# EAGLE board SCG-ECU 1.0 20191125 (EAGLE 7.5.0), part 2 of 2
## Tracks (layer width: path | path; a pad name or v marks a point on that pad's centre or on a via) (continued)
N$3 (continued)
  Top 0.61: R67.1 79.63,102.01 80.16,101.47 80.16,100.03 U$9.5
N$4  (via drill 0.5)
  other vias: 11.05,95
N$5
  Top 0.61: R68.1 76.86,102.23 77.57,101.52 77.57,100.03 U$9.7
N$6
  Top 0.61: R35.1 64.54,101.91 65.02,101.42 U$11.5
N$7  (via drill 0.5)
  other vias: 12.32,95
N$8
  Top 0.61: R36.1 61.85,102.16 62.48,101.52 U$11.7
N$9
  Top 0.254: Q2.1 47.76,58.41 R50.1 R61.1
N$10  (via drill 0.5)
  other vias: 13.59,95
N$11
  Top 0.254: Q3.1 46.56,48.35 R62.1 R69.1
N$12
  Top 0.305: U1.8 64.24,77.39 65,76.63 69.64,76.63 R22.1
N$13
  Top 0.305: R79.2 R78.1 50.67,6.35 52.07,7.75 52.07,10.54 52.96,11.43 U3.10
N$14  (via drill 0.5)
  other vias: 14.86,95
N$15
  Top 0.305: R77.2 R76.1 44.83,15.62 46.48,13.97 U3.3
N$16
  Top 0.305: R30.1 73.73,87.22 LED1.A
N$17
  Top 0.305: R117.2 R116.1 45.59,8.64 46.23,9.27 46.23,10.54 47.12,11.43 U3.5
N$18
  Top 0.305: R84.2 15.77,103.43 16.51,102.49 LED9.A
N$19
  Top 0.254: C6.+ 49.15,91.44 49.15,91.19
  Top 0.813: STEPSTICK-X.VMOT 44.96,101.73 46.61,100.08 48.61,100.08 L2.1 48.64,91.7 49.15,91.19 46.7,91.19 C4.1
N$20
  Top 0.305: R100.2 118.87,88.27 117.86,87.25 LED11.A
N$21
  Top 0.305: R138.2 16.76,73.91 17.78,72.9 LED15.A
N$22
  Top 0.305: R86.2 118.75,103.76 117.86,102.87 LED10.A
N$23  (via drill 0.5)
  other vias: 14.86,93.73
N$24  (via drill 0.5)
  other vias: 13.59,93.73
N$25
  Top 0.305: R31.1 82.61,86.97 LED2.A
N$26  (via drill 0.5)
  other vias: 12.32,93.73
N$27
  Top 0.254: R46.1 49.09,36.76 48.77,37.08 C19.1 R47.2 | 47.75,39.69 49.4,39.69
  Top 0.406: 47.75,39.69 R47.2 | 49.4,39.69 R48.1
N$28  (via drill 0.5)
  other vias: 11.05,93.73
N$29
  Top 0.254: R74.1 R71.1 Q4.1
N$30  (via drill 0.5)
  other vias: 11.05,92.46
N$31
  Top 0.305: R102.2 17.02,30.23 17.78,29.46 LED12.A
N$32
  Top 0.305: C17.2 115.47,12.55 114.55,13.46 114.55,15.11 113.79,15.88 109.35,15.88 108.58,15.11 PS1.4 106.52,14.19 106.05,13.72 104.48,13.72 R45.1
N$33  (via drill 0.5)
  other vias: 12.32,92.46
N$34
  Top 0.305: R140.2 118.87,44.7 117.98,43.82 LED16.A
N$35
  Top 0.305: R57.1 105.54,88.58 105.54,87.88 104.39,86.74 C25.2 101.6,86.68 101.6,85.98 100.35,84.73 U$10.9
N$36
  Top 0.305: R60.1 89.66,88.84 89.66,88.01 90.68,86.99 C26.1 93.6,86.93 93.6,86.11 94.97,84.73 U$10.16
N$37
  Top 0.305: R59.1 C26.2 96.08,86.48 U$10.15
N$38
  Top 0.305: 99.25,88.13 R28.1 C25.1 99.25,86.23 U$10.10
N$39
  Top 0.61: R106.1 38.53,80.39 38,79.86 37.13,79.86 36.17,78.89 36.17,77.35 U$25.5
N$40
  Top 0.61: R107.1 30.2,80.29 30.73,79.76 32.56,79.76 33.63,78.69 33.63,77.35 U$25.7
N$41
  Top 0.305: R25.1 R60.2
N$42
  Top 0.61: R110.1 56.61,80.39 56.08,79.86 55.32,79.86 54.25,78.79 54.25,77.35 U$26.5
N$43
  Top 0.61: R111.1 48.06,80.41 48.62,79.86 50.65,79.86 51.71,78.79 51.71,77.35 U$26.7
N$44
  Top 0.254: R112.1 28.36,73 LED20.A
N$45
  Top 0.254: R113.1 40.47,73.15 LED21.A
N$46
  Top 0.254: R114.1 46.14,73.05 LED22.A
N$47
  Top 0.254: R115.1 58.48,73.08 LED23.A
N$48  (via drill 0.5)
  other vias: 14.86,92.46
N$49
  Top 0.305: R65.2 103.41,74.92 LED7.C
N$50
  Top 0.305: R64.2 91.58,75.06 LED6.C
N$51
  Top 0.305: 12V.A R23.1
N$52  (via drill 0.5)
  other vias: 13.59,92.46
N$53  (via drill 0.5)
  other vias: 11.05,80.39
N$54
  Top 0.305: R130.1 96.97,35.2 5V.A
N$55
  Top 0.305: R59.2 R26.1
N$56
  Top 0.305: R27.1 R57.2
N$57
  Top 0.305: R56.1 R28.2
N$58
  Top 0.305: U2.3 91.44,11.18 91.95,10.67 R123.2 R122.1
N$59
  Top 0.305: R118.1 R119.2 44.83,20.19 47.12,17.91 49.91,17.91 51.31,16.51 51.31,14.99 52.32,13.97 U3.12
N$60  (via drill 0.5)
  other vias: 12.32,80.39
N$61  (via drill 0.5)
  other vias: 13.59,80.39
N$62  (via drill 0.5)
  other vias: 14.86,80.39
N$63  (via drill 0.5)
  other vias: 14.86,79.12
N$64  (via drill 0.5)
  other vias: 13.59,79.12
N$65
  Top 0.305: R125.2 R124.1 92.5,19.91 88.27,19.91 87.2,20.98 80.03,20.98 79.43,20.37 79.43,17.83 79.83,17.42 81.2,17.42 82.32,16.31 82.32,14.07 81.97,13.72 U2.10
N$66
  Top 0.305: R127.2 R126.1 88.77,13.08 88.14,13.72 U2.5
N$67
  Top 0.305: U2.12 81.41,11.18 82.42,10.16 82.42,7.11 83.44,6.1 89.73,6.1 R129.2 R128.1
N$68
  Top 0.305: R122.2 96.27,8.2 JP1.1
N$69
  Top 0.305: U2.2 U2.1 JP2.1
N$70
  Top 0.305: R126.2 JP3.1
N$71
  Top 0.305: U2.6 U2.7 88.27,18.29 JP4.1
N$72
  Top 0.305: R120.1 58.61,87.22 LED3.A
N$73
  Top 0.305: R121.1 67.37,86.97 LED4.A
N$74
  Top 0.305: R131.2 91.57,69.85 90.81,69.09 90.81,65.15 91.44,64.52 93.02,64.52 U$18.3
N$75
  Top 1.27: D16.C 83.29,50.7 | 83.29,50.7 L3.2 | 83.29,50.7 83.29,50.19 82.42,49.33 81.25,49.33 80.09,48.16 80.09,46.28 L1.2
N$76
  Top 1.27: U$28.1 91.26,30.99 89.89,32.36 88.3,32.36 C45.+ 87.71,32.91 87.71,33.12 85.57,35.26 82.32,35.26 80.11,37.47 L1.1
N$77
  Top 0.305: 5V1.A 102.35,21.23 R132.1
N$78  (via drill 0.7)
  Top 1.27: U$27.1 98.07,39.75 | 98.07,39.75 99.11,39.75 100.71,38.15 102.35,38.15 C28.+ | L3.1 91.39,50.01 v93.45,47.96 | v97.66,42.42 97.66,40.16 98.07,39.75
  Bottom 1.27: v93.45,47.96 93.45,46.63 v97.66,42.42
N$79
  Top 0.305: R133.2 17.27,44.7 18.03,43.94 LED13.A
N$80  (via drill 0.5)
  other vias: 12.32,79.12
N$81
  Top 0.305: R137.1 30.06,29.78 30.81,30.53 31.82,30.53 3V3.A
N$82  (via drill 0.5)
  other vias: 11.05,79.12
N$83
  Top 0.305: R135.2 17.02,59.18 17.91,58.29 LED14.A
N$84
  Top 0.305: R142.2 118.87,30.35 117.98,29.46 LED17.A
N$85  (via drill 0.5)
  other vias: 11.05,77.85
N$86  (via drill 0.5)
  other vias: 12.32,77.85
N$87
  Top 0.305: R144.2 118.87,59.18 118.11,58.42 LED18.A
N$88  (via drill 0.5)
  other vias: 13.59,77.85
N$89  (via drill 0.5)
  other vias: 14.86,77.85
N$90  (via drill 0.5)
  other vias: 11.05,65.79
N$91
  Top 0.254: 47.4,63.74 R72.1 | R72.1 R73.1 | Q1.1 47.75,63.39 R72.1
N$92  (via drill 0.5)
  other vias: 12.32,65.79
N$93  (via drill 0.5)
  other vias: 13.59,65.79
N$94  (via drill 0.5)
  other vias: 14.86,65.79
N$95  (via drill 0.5)
  other vias: 14.86,64.52
N$96  (via drill 0.5)
  other vias: 13.59,64.52
N$97  (via drill 0.5)
  other vias: 12.32,64.52
N$98  (via drill 0.5)
  other vias: 11.05,64.52
N$99  (via drill 0.5)
  other vias: 11.05,63.25
N$100  (via drill 0.5)
  other vias: 12.32,63.25
N$101  (via drill 0.5)
  other vias: 13.59,63.25
N$102  (via drill 0.5)
  other vias: 14.86,63.25
N$103  (via drill 0.5)
  other vias: 11.05,51.18
N$104  (via drill 0.5)
  other vias: 12.32,51.18
N$105  (via drill 0.5)
  other vias: 13.59,51.18
N$106  (via drill 0.5)
  other vias: 14.86,51.18
N$107  (via drill 0.5)
  other vias: 14.86,49.91
N$108  (via drill 0.5)
  other vias: 13.59,49.91
N$109  (via drill 0.5)
  other vias: 12.32,49.91
N$110  (via drill 0.5)
  other vias: 11.05,49.91
N$111  (via drill 0.5)
  other vias: 11.05,48.64
N$112  (via drill 0.5)
  other vias: 12.32,48.64
N$113  (via drill 0.5)
  other vias: 13.59,48.64
N$114  (via drill 0.5)
  other vias: 14.86,48.64
N$115  (via drill 0.5)
  other vias: 11.05,36.58
N$116  (via drill 0.5)
  other vias: 12.32,36.58
N$117  (via drill 0.5)
  other vias: 13.59,36.58
N$118  (via drill 0.5)
  other vias: 14.86,36.58
N$119  (via drill 0.5)
  other vias: 14.86,35.31
N$120  (via drill 0.5)
  other vias: 13.59,35.31
N$121  (via drill 0.5)
  other vias: 12.32,35.31
N$122  (via drill 0.5)
  other vias: 11.05,35.31
N$123  (via drill 0.5)
  other vias: 11.05,34.04
N$124  (via drill 0.5)
  other vias: 12.32,34.04
N$125  (via drill 0.5)
  other vias: 13.59,34.04
N$126  (via drill 0.5)
  other vias: 14.86,34.04
N$127  (via drill 0.5)
  other vias: 11.05,21.97
N$128  (via drill 0.5)
  other vias: 12.32,21.97
N$129  (via drill 0.5)
  other vias: 13.59,21.97
N$130  (via drill 0.5)
  other vias: 14.86,21.97
N$131  (via drill 0.5)
  other vias: 14.86,20.7
N$132  (via drill 0.5)
  other vias: 13.59,20.7
N$133  (via drill 0.5)
  other vias: 12.32,20.7
N$134  (via drill 0.5)
  other vias: 11.05,20.7
N$135  (via drill 0.5)
  other vias: 11.05,19.43
N$136  (via drill 0.5)
  other vias: 12.32,19.43
N$137  (via drill 0.5)
  other vias: 13.59,19.43
N$138  (via drill 0.5)
  other vias: 14.86,19.43
N$139  (via drill 0.5)
  other vias: 83.44,46.74
N$140  (via drill 0.5)
  other vias: 84.71,46.74
N$141  (via drill 0.5)
  other vias: 85.98,46.74
N$142  (via drill 0.5)
  other vias: 87.25,46.74
N$143  (via drill 0.5)
  other vias: 88.52,46.74
N$144  (via drill 0.5)
  other vias: 89.79,46.74
N$145  (via drill 0.5)
  other vias: 89.79,45.47
N$146  (via drill 0.5)
  other vias: 88.52,45.47
N$147  (via drill 0.5)
  other vias: 87.25,45.47
N$148  (via drill 0.5)
  other vias: 85.98,45.47
N$149  (via drill 0.5)
  other vias: 84.71,45.47
N$150  (via drill 0.5)
  other vias: 83.44,45.47
N$151  (via drill 0.5)
  other vias: 83.44,44.2
N$152  (via drill 0.5)
  other vias: 84.71,44.2
N$153  (via drill 0.5)
  other vias: 85.98,44.2
N$154  (via drill 0.5)
  other vias: 87.25,44.2
N$155  (via drill 0.5)
  other vias: 88.52,44.2
N$156  (via drill 0.5)
  other vias: 89.79,44.2
N$157  (via drill 0.5)
  other vias: 89.79,42.93
N$158  (via drill 0.5)
  other vias: 88.52,42.93
N$159  (via drill 0.5)
  other vias: 87.25,42.93
N$160  (via drill 0.5)
  other vias: 85.98,42.93
N$161  (via drill 0.5)
  other vias: 84.71,42.93
N$162  (via drill 0.5)
  other vias: 83.44,42.93
N$163  (via drill 0.5)
  other vias: 83.44,41.66
N$164  (via drill 0.5)
  other vias: 84.71,41.66
N$165  (via drill 0.5)
  other vias: 85.98,41.66
N$166  (via drill 0.5)
  other vias: 87.25,41.66
N$167  (via drill 0.5)
  other vias: 88.52,41.66
N$168  (via drill 0.5)
  other vias: 89.79,41.66
N$169  (via drill 0.5)
  other vias: 89.79,40.39
N$170  (via drill 0.5)
  other vias: 88.52,40.39
N$171  (via drill 0.5)
  other vias: 87.25,40.39
N$172  (via drill 0.5)
  other vias: 85.98,40.39
N$173  (via drill 0.5)
  other vias: 84.71,40.39
N$174  (via drill 0.5)
  other vias: 83.44,40.39
N$175  (via drill 0.5)
  other vias: 83.44,39.12
N$176  (via drill 0.5)
  other vias: 84.71,39.12
N$177  (via drill 0.5)
  other vias: 85.98,39.12
N$178  (via drill 0.5)
  other vias: 87.25,39.12
N$179  (via drill 0.5)
  other vias: 88.52,39.12
N$180  (via drill 0.5)
  other vias: 89.79,39.12
N$181  (via drill 0.5)
  other vias: 89.79,37.85
N$182  (via drill 0.5)
  other vias: 88.52,37.85
N$183  (via drill 0.5)
  other vias: 87.25,37.85
N$184  (via drill 0.5)
  other vias: 85.98,37.85
N$185  (via drill 0.5)
  other vias: 84.71,37.85
N$186  (via drill 0.5)
  other vias: 83.44,37.85
N$187  (via drill 0.5)
  other vias: 101.22,32.77
N$188  (via drill 0.5)
  other vias: 102.49,32.77
N$189  (via drill 0.5)
  other vias: 103.76,32.77
N$190  (via drill 0.5)
  other vias: 105.03,32.77
N$191  (via drill 0.5)
  other vias: 106.3,32.77
N$192  (via drill 0.5)
  other vias: 107.57,32.77
N$193  (via drill 0.5)
  other vias: 107.57,31.5
N$194  (via drill 0.5)
  other vias: 106.3,31.5
N$195  (via drill 0.5)
  other vias: 105.03,31.5
N$196  (via drill 0.5)
  other vias: 103.76,31.5
N$197  (via drill 0.5)
  other vias: 102.49,31.5
N$198  (via drill 0.5)
  other vias: 101.22,31.5
N$199  (via drill 0.5)
  other vias: 101.22,30.23
N$200  (via drill 0.5)
  other vias: 102.49,30.23
N$201  (via drill 0.5)
  other vias: 103.76,30.23
N$202  (via drill 0.5)
  other vias: 105.03,30.23
N$203  (via drill 0.5)
  other vias: 106.3,30.23
N$204  (via drill 0.5)
  other vias: 107.57,30.23
N$205  (via drill 0.5)
  other vias: 107.57,28.96
N$206  (via drill 0.5)
  other vias: 106.3,28.96
N$207  (via drill 0.5)
  other vias: 105.03,28.96
N$208  (via drill 0.5)
  other vias: 103.76,28.96
N$209  (via drill 0.5)
  other vias: 102.49,28.96
N$210  (via drill 0.5)
  other vias: 101.22,28.96
N$211  (via drill 0.5)
  other vias: 101.22,27.69
N$212  (via drill 0.5)
  other vias: 102.49,27.69
N$213  (via drill 0.5)
  other vias: 103.76,27.69
N$214  (via drill 0.5)
  other vias: 105.03,27.69
N$215  (via drill 0.5)
  other vias: 106.3,27.69
N$216  (via drill 0.5)
  other vias: 107.57,27.69
N$217  (via drill 0.5)
  other vias: 107.57,26.42
N$218  (via drill 0.5)
  other vias: 106.3,26.42
N$219  (via drill 0.5)
  other vias: 105.03,26.42
N$220  (via drill 0.5)
  other vias: 103.76,26.42
N$221  (via drill 0.5)
  other vias: 102.49,26.42
N$222  (via drill 0.5)
  other vias: 101.22,26.42
N$223  (via drill 0.5)
  other vias: 101.22,25.15
N$224  (via drill 0.5)
  other vias: 102.49,25.15
N$225  (via drill 0.5)
  other vias: 103.76,25.15
N$226  (via drill 0.5)
  other vias: 105.03,25.15
N$227  (via drill 0.5)
  other vias: 106.3,25.15
N$228  (via drill 0.5)
  other vias: 107.57,25.15
N$229  (via drill 0.5)
  other vias: 107.57,23.88
N$230  (via drill 0.5)
  other vias: 106.3,23.88
N$231  (via drill 0.5)
  other vias: 105.03,23.88
N$232  (via drill 0.5)
  other vias: 103.76,23.88
N$233  (via drill 0.5)
  other vias: 102.49,23.88
N$234  (via drill 0.5)
  other vias: 101.22,23.88
N$235  (via drill 0.5)
  other vias: 85.34,67.69
N$236  (via drill 0.5)
  other vias: 86.61,67.69
N$237  (via drill 0.5)
  other vias: 87.88,67.69
N$238  (via drill 0.5)
  other vias: 89.15,67.69
N$239  (via drill 0.5)
  other vias: 89.15,66.42
N$240  (via drill 0.5)
  other vias: 87.88,66.42
N$241  (via drill 0.5)
  other vias: 86.61,66.42
N$242  (via drill 0.5)
  other vias: 85.34,66.42
N$243  (via drill 0.5)
  other vias: 85.34,65.15
N$244  (via drill 0.5)
  other vias: 86.61,65.15
N$245  (via drill 0.5)
  other vias: 87.88,65.15
N$246  (via drill 0.5)
  other vias: 89.15,65.15
N$247  (via drill 0.5)
  other vias: 89.15,63.88
N$248  (via drill 0.5)
  other vias: 87.88,63.88
N$249  (via drill 0.5)
  other vias: 86.61,63.88
N$250  (via drill 0.5)
  other vias: 85.34,63.88
N$251  (via drill 0.5)
  other vias: 86.61,62.61
N$252  (via drill 0.5)
  other vias: 87.88,62.61
N$253  (via drill 0.5)
  other vias: 89.15,62.61
N$254  (via drill 0.5)
  other vias: 120.27,95.63
N$255  (via drill 0.5)
  other vias: 121.54,95.63
N$256  (via drill 0.5)
  other vias: 122.81,95.63
N$257  (via drill 0.5)
  other vias: 124.08,95.63
N$258  (via drill 0.5)
  other vias: 124.08,94.36
N$259  (via drill 0.5)
  other vias: 122.81,94.36
N$260  (via drill 0.5)
  other vias: 121.54,94.36
N$261  (via drill 0.5)
  other vias: 120.27,94.36
N$262  (via drill 0.5)
  other vias: 120.27,93.09
N$263  (via drill 0.5)
  other vias: 121.54,93.09
N$264  (via drill 0.5)
  other vias: 122.81,93.09
N$265  (via drill 0.5)
  other vias: 124.08,93.09
N$266  (via drill 0.5)
  other vias: 120.27,80.39
N$267  (via drill 0.5)
  other vias: 121.54,80.39
N$268  (via drill 0.5)
  other vias: 122.81,80.39
N$269  (via drill 0.5)
  other vias: 124.08,80.39
N$270  (via drill 0.5)
  other vias: 124.08,79.12
N$271  (via drill 0.5)
  other vias: 122.81,79.12
N$272  (via drill 0.5)
  other vias: 121.54,79.12
N$273  (via drill 0.5)
  other vias: 120.27,79.12
N$274  (via drill 0.5)
  other vias: 120.27,77.85
N$275  (via drill 0.5)
  other vias: 121.54,77.85
N$276  (via drill 0.5)
  other vias: 122.81,77.85
N$277  (via drill 0.5)
  other vias: 124.08,77.85
N$278  (via drill 0.5)
  other vias: 120.9,65.79
N$279  (via drill 0.5)
  other vias: 122.17,65.79
N$280  (via drill 0.5)
  other vias: 123.44,65.79
N$281  (via drill 0.5)
  other vias: 124.71,65.79
N$282  (via drill 0.5)
  other vias: 124.71,64.52
N$283  (via drill 0.5)
  other vias: 123.44,64.52
N$284  (via drill 0.5)
  other vias: 122.17,64.52
N$285  (via drill 0.5)
  other vias: 120.9,64.52
N$286  (via drill 0.5)
  other vias: 120.9,63.25
N$287  (via drill 0.5)
  other vias: 122.17,63.25
N$288  (via drill 0.5)
  other vias: 123.44,63.25
N$289  (via drill 0.5)
  other vias: 124.71,63.25
N$290  (via drill 0.5)
  other vias: 120.9,50.55
N$291  (via drill 0.5)
  other vias: 122.17,50.55
N$292  (via drill 0.5)
  other vias: 123.44,50.55
N$293  (via drill 0.5)
  other vias: 124.71,50.55
N$294  (via drill 0.5)
  other vias: 124.71,49.28
N$295  (via drill 0.5)
  other vias: 123.44,49.28
N$296  (via drill 0.5)
  other vias: 122.17,49.28
N$297  (via drill 0.5)
  other vias: 120.9,49.28
N$298  (via drill 0.5)
  other vias: 120.9,48.01
N$299  (via drill 0.5)
  other vias: 122.17,48.01
N$300  (via drill 0.5)
  other vias: 123.44,48.01
N$301  (via drill 0.5)
  other vias: 124.71,48.01
N$302  (via drill 0.5)
  other vias: 120.9,36.58
N$303  (via drill 0.5)
  other vias: 122.17,36.58
N$304  (via drill 0.5)
  other vias: 123.44,36.58
N$305  (via drill 0.5)
  other vias: 124.71,36.58
N$306  (via drill 0.5)
  other vias: 124.71,35.31
N$307  (via drill 0.5)
  other vias: 123.44,35.31
N$308  (via drill 0.5)
  other vias: 122.17,35.31
N$309  (via drill 0.5)
  other vias: 120.9,35.31
N$310  (via drill 0.5)
  other vias: 120.9,34.04
N$311  (via drill 0.5)
  other vias: 122.17,34.04
N$312  (via drill 0.5)
  other vias: 123.44,34.04
N$313  (via drill 0.5)
  other vias: 124.71,34.04
N$314  (via drill 0.5)
  other vias: 120.9,21.97
N$315  (via drill 0.5)
  other vias: 122.17,21.97
N$316  (via drill 0.5)
  other vias: 123.44,21.97
N$317  (via drill 0.5)
  other vias: 124.71,21.97
N$318  (via drill 0.5)
  other vias: 124.71,20.7
N$319  (via drill 0.5)
  other vias: 123.44,20.7
N$320  (via drill 0.5)
  other vias: 122.17,20.7
N$321  (via drill 0.5)
  other vias: 120.9,20.7
N$322  (via drill 0.5)
  other vias: 120.9,19.43
N$323  (via drill 0.5)
  other vias: 122.17,19.43
N$324  (via drill 0.5)
  other vias: 123.44,19.43
N$325  (via drill 0.5)
  other vias: 124.71,19.43
N$326
  Top 0.406: R107.2 27.4,83.46 28.63,84.68 32.79,84.68 JP15.1
N$327
  Top 0.406: JP16.1 45.54,80.85 R111.2
N$328
  Top 0.406: R106.2 41.33,81.99 40.46,82.85 JP18.2
N$329
  Top 0.406: R110.2 59.41,82.55 58.6,83.36 52.09,83.36 JP17.2
N$330
  pour Top: 112.65,89.92 113.92,89.92 113.92,88.65 112.65,88.65
N$331
  pour Top: 112.65,74.68 113.92,74.68 113.92,73.41 112.65,73.41
N$332
  pour Top: 112.65,48.01 113.92,48.01 113.92,46.74 112.65,46.74
N$333
  pour Top: 112.65,32.77 113.92,32.77 113.92,31.5 112.65,31.5
N$334
  pour Top: 112.65,18.8 113.92,18.8 113.92,17.53 112.65,17.53
N$335
  pour Bottom: 23.75,53.09 25.02,53.09 25.02,51.82 23.75,51.82
N$336
  pour Bottom: 23.75,45.47 25.02,45.47 25.02,44.2 23.75,44.2
N$337
  pour Bottom: 23.75,31.5 25.02,31.5 25.02,32.77 23.75,32.77
N$338
  Top 0.305: JP20.3 JP21.1
N$339
  Top 0.305: JP20.2 102.5,16.92 R45.2 102.48,13.67 101.52,13.67 100.64,12.78 C18.2
O2  (via drill 0.5)
  Top 0.254: R21.2 81.6,79.5 D2.C 77.4,79.5 D1.A
  Top 0.305: R116.2 39.12,8.64 v38.23,9.53 | v75.82,81.53 75.69,81.53 74.8,80.64 D1.A | v64.44,55.07 66.37,55.07 66.93,55.63 66.93,66.7 v67.49,67.26
  Top 0.406: 79.82,79.18 D2.C | 77.4,79.5 C2.1
  Bottom 0.305: v38.23,9.53 49.15,9.53 50.29,8.38 57.66,8.38 59.44,6.6 62.36,6.6 66.93,11.18 66.93,20.22 67.39,20.68 67.39,21.74 66.98,22.15 66.98,42.57 63.63,45.92 63.63,52.32 64.39,53.09 64.39,55.02 v64.44,55.07 | v75.82,81.53 74.6,81.53 68.76,75.69 68.76,68.63 67.49,67.36 v67.49,67.26
O2_2
  Top 0.254: D17.C D15.A
  Top 0.305: R128.2 93.15,2.16 113.67,2.16 115.06,3.56 115.06,5.71 115.82,6.48 115.82,9.02 116.84,10.03 D17.C 118.49,10.09 118.18,10.09 | D15.A 122.42,10.03 R37.2 122.75,9.7 C37.1
O2_2_CPU  (via drill 0.5)
  Top 0.305: U2.13 U2.14 80.64,7.52 79.02,5.89 63.42,5.89 61.85,7.47 61.85,11.43 65.28,14.86 65.28,18.29 64.14,19.43 62.48,19.43 61.85,20.07 61.85,21.21 61.09,21.97 59.69,21.97 59.18,22.48 59.18,24.26 58.55,24.89 58.55,30.73 v58.09,31.19
  Bottom 0.305: v58.09,31.19 57.99,31.19 57.78,31.39 57.78,45.16 58.75,46.13 60.55,46.13 U$1.A22/DAC1
O2_2_SENSOR
  Top 0.254: R37.1 C36.1
  Top 0.406: C36.1 125.66,11.75 127.38,13.46 127.38,17.14 131.7,21.46 131.7,38.23 132.97,39.5 132.97,108.46 126.11,115.32 126.11,116.84 123.7,119.25 105.87,119.25 U$17.36
O2_CPU  (via drill 0.5)
  Top 0.305: U3.7 U3.6 50.04,10.16 v51.05,9.14
  Bottom 0.305: v51.05,9.14 51.18,9.27 63.75,9.27 65.91,11.43 65.91,20.57 63.37,23.11 63.37,24.23 62.56,25.04 62.56,26.21 61.8,26.97 61.8,31.45 61.09,32.16 58.8,32.16 58.4,32.56 58.4,43.94 59.26,44.81 61.34,44.81 61.85,45.31 61.85,47.37 U$1.21/DAC0
O2_SENSOR
  Top 0.254: C1.1 R21.1
  Top 0.305: C1.1 84.33,76.71
  Top 0.406: 84.33,76.71 85.72,76.71 87.2,78.18 87.2,111.46 U$17.45
RST_CPU  (via drill 0.5)
  Top 0.254: D13.A 70.61,32.26 70.18,32.69 68.37,32.69 R49.2 C21.1
  Top 0.305: C21.1 64.65,32.71 64.08,33.27 64.08,36.73 v65.96,38.61
  Bottom 0.305: v65.96,38.61 65.56,39.01 65.56,43.18 63.07,45.67 63.07,53.67 U$1.RESET
RX5  (via drill 0.5)
  Top 0.305: v71.04,80.97 71.04,81.03 71.14,81.13 71.14,81.23 71.25,81.23 71.25,109.17 77.5,115.42 85.37,115.42 U$17.31
  Bottom 0.305: v71.04,80.97 70.74,80.67 70.74,78.59 61.8,69.65 61.8,65.43 60.58,64.21 U$1.34/A15
RX_CPU  (via drill 0.5)
  Top 0.305: v81,84.48 82.93,84.48 84.45,86 84.45,98.96 v83.39,100.02 | v68.86,67.26 69.93,66.19 69.93,55.93 69.06,55.07 67.54,55.07 66.93,54.46 66.93,44.78 v68.4,43.31
  Bottom 0.305: U$1.0/RX 72.95,10.54 70.08,13.41 70.08,16.76 69.06,17.78 69.06,26.36 68.33,27.1 68.33,43.48 v68.4,43.31 | v81,84.48 80.9,84.38 80.34,84.38 76.28,80.31 76.28,80.26 74.24,80.26 69.37,75.39 69.37,67.72 68.91,67.26 v68.86,67.26 | v83.39,100.02 83.39,108.56 81.81,110.13 81.81,114.98 U$17.29
SCK2
  Top 0.305: U$1.53 62.79,46.1 61.54,47.35 JP5.1
SCL  (via drill 0.5)
  Top 0.305: v57.33,92.51 56.92,92.1 56.92,86.51 v55.04,84.63 | U$1.19/A5/SCL 61.72,25.78 v63.02,27.08 | v51.49,44.35 51.94,44.81 62.51,44.81 64.44,42.88 v64.44,42.72
  Bottom 0.305: v57.33,92.51 57.33,114.67 U$17.14 | v63.02,27.08 65,29.06 65,42.16 v64.44,42.72 | v51.49,44.35 50.55,45.29 50.55,69.34 51.69,70.48 53.85,70.48 55.4,72.03 55.4,84.28 v55.04,84.63
SDA  (via drill 0.5)
  Top 0.305: v55.75,93.22 56.31,92.66 56.31,86.87 55.35,85.9 v53.98,85.9 | U$1.18/A4/SDA 62.64,28.32 v62.66,28.3 | v49.86,43.84 49.86,43.74 50.16,43.43 58.14,43.43 59.31,42.27 v63.12,42.27
  Bottom 0.305: v55.75,93.22 56.36,93.22 56.77,93.62 56.77,113.79 55.24,115.32 52.65,115.32 51.94,116.03 51.94,116.72 U$17.13 | v63.12,42.27 64.34,41 64.34,29.97 v62.66,28.3 | v49.86,43.84 49.91,43.89 49.91,69.6 51.44,71.12 53.59,71.12 54.81,72.34 54.84,72.34 54.84,83.57 53.98,84.43 v53.98,85.9
STEP_1A
  Bottom 1.27: U$17.20 28.61,106.64 32,103.25 32,101.75 STEPSTICK-X.1A
STEP_1B
  Bottom 1.27: U$17.21 31.94,106.36 34.54,103.76 34.54,101.75 STEPSTICK-X.1B
STEP_2A
  Bottom 1.27: U$17.22 35.27,105.95 37.08,104.14 37.08,101.75 STEPSTICK-X.2A
STEP_2B
  Bottom 1.27: U$17.23 38.6,105.55 39.62,104.52 39.62,101.75 STEPSTICK-X.2B
STP  (via drill 0.5)
  Top 0.305: v60.53,84.33 60.58,84.28 60.73,84.28 61.59,83.41 61.59,71.02 59.77,69.19 v59.71,69.19
  Bottom 0.305: U$1.35/A16 60.15,61.34 59.05,62.43 59.05,68.53 v59.71,69.19 | v60.53,84.33 60.53,87.02 57.73,89.81 50.01,89.81 47.57,92.25 30.86,92.25 29.44,90.83 29.44,89.08
  Bottom 0.406: 29.44,89.08 STEPSTICK-X.SPT
TACHO
  Top 0.254: Q4.3 42.31,51.4 R75.1
  Top 0.406: Q4.3 39.98,54.64 39.5,55.12 39.5,59.05 35.18,63.37 30.73,63.37 24.26,69.85 24.26,74.55 23.37,75.44 23.37,112.78 22.73,113.41 20.83,113.41 18.67,115.57 18.67,116.7 U$17.3
TACHO_CPU  (via drill 0.5)
  Top 0.305: R71.2 50.7,53.7 v52.09,52.3
  Bottom 0.305: U$1.21/A7 60.58,20.83 62.1,22.35 62.1,23.62 61.21,24.51 59.56,24.51 57.89,26.19 57.89,29.01 56.46,30.43 56.46,38.76 53.87,41.35 53.87,45.87 51.84,47.9 51.84,51.87 52.09,52.12 v52.09,52.3
TPS  (via drill 0.5)
  Top 0.254: D10.C 53.27,24.36 D9.A
  Top 0.305: C14.1 51.04,24.3 | R118.2 41.47,24.45 v41.15,24.76 | v53.47,26.42 53.47,24.56 D9.A
  Top 0.406: 51.1,22.01 C14.1 | 51.04,24.3 D10.C 51.1,26.46 R44.2
  Bottom 0.305: v41.15,24.76 51.82,24.76 v53.47,26.42
TPS_CPU
  Top 0.305: U3.14 U3.13 54.86,15.24 55.75,14.35 56.9,14.35 57.94,15.39 57.94,23.98 57.23,24.69 57.23,32.11 58.52,33.4 U$1.16/A2
TPS_SIGNAL  (via drill 0.5)
  Top 0.305: C13.1 47.8,28.42 v46.56,29.67
  Top 0.406: R44.1 C13.1
  Bottom 0.305: U$17.11 43.46,114.95 43.46,100.69 42.49,99.72 26.95,99.72 25.68,98.45 25.68,87.88 26.64,86.92 54.84,86.92 56.01,85.75 56.01,71.75 54.1,69.85 51.94,69.85 51.18,69.09 51.18,46.03 52.55,44.65 52.55,31.65 51.03,30.12 47.02,30.12 v46.56,29.67
TX5  (via drill 0.5)
  Top 0.305: v70.23,81.99 70.43,82.19 70.23,82.19 70.13,82.09 70.13,84.58 70.64,85.09 70.64,109.78 78.97,118.11 88.72,118.11 90.04,116.79 U$17.32
  Bottom 0.305: U$1.33/A14 60.58,69.24 70.08,78.74 70.08,81.84 v70.23,81.99
TX_CPU  (via drill 0.5)
  Top 0.305: v80.64,83.31 82.88,83.31 85.11,85.55 85.11,100.48 v84.51,101.09 | v71.86,48.11 71.86,51.33 70.74,52.45 69.98,52.45 69.47,52.96 69.47,54.51 70.59,55.63 70.59,66.95 v70.28,67.26
  Bottom 0.305: U$1.1/TX 71.53,13.08 70.79,13.82 70.79,17.12 69.83,18.08 69.83,26.52 68.96,27.38 68.96,41.53 71.86,44.43 v71.86,48.11 | v80.64,83.31 80.24,83.31 76.58,79.65 74.55,79.65 70.03,75.13 70.03,71.83 70.54,71.32 70.54,67.61 70.28,67.36 v70.28,67.26 | v84.51,101.09 84.51,115.62 U$17.30
UD+  (via drill 0.5)
  Top 0.305: v83.54,81.58 83.54,81.99 86.33,84.78 86.33,84.84 86.39,84.89 86.39,110.18 85.42,111.15 85.42,112.88 86.03,113.49 95.53,113.49 96.75,114.71 96.75,116.7 U$17.34 | v73.36,45.95 73.79,46.38 73.79,49.53 74.55,50.29 74.55,64.46 73.79,65.23 73.79,66.45 v72.95,67.28
  Bottom 0.305: U$1.UD+ 72.19,19.43 71.25,20.37 71.25,26.87 70.33,27.79 70.33,41.12 73.36,44.15 v73.36,45.95 | v83.54,81.58 83.19,81.23 79.93,81.23 77.09,78.38 75.01,78.38 71.37,74.75 71.4,74.73 71.4,72.39 72.95,70.84 v72.95,67.28
UD-  (via drill 0.5)
  Top 0.305: v81.46,82.14 82.68,82.14 85.78,85.24 85.78,109.83 84.66,110.95 84.66,113.13 85.67,114.15 92.23,114.15 93.4,115.32 93.4,116.72 U$17.33 | v72.87,47.12 72.87,51.97 72.01,52.83 72.01,54.61 72.64,55.25 73.41,55.25 73.91,55.75 73.91,64.08 73.08,64.92 73.08,65.86 v71.65,67.28
  Bottom 0.305: U$1.UD- 72.14,16.89 70.59,18.44 70.59,26.67 69.67,27.58 69.67,41.35 72.52,44.2 72.52,46.61 72.87,46.97 v72.87,47.12 | v81.46,82.14 81.36,82.04 79.88,82.04 76.83,78.99 74.75,78.99 70.69,74.93 70.74,74.88 70.74,72.08 71.65,71.17 v71.65,67.28
VIN  (via drill 0.7)
  Top 0.305: U$18.1 93.09,62.87 94.36,62.87 94.36,63.75 91.95,63.75 91.95,62.74 94.36,62.74 94.36,63.25 94.11,63.25 94.11,63.5 93.85,63.5 93.85,63.25 93.85,63.12 93.6,63.12 | U$18.2 93.6,63.73 93.6,63.12 | 93.6,63.12 93.34,63.12 93.34,63.5 93.09,63.5 93.09,63.12 92.84,63.12 92.84,63.5 92.58,63.5 92.58,63.25 92.33,63.25 92.33,63.5 92.08,63.5 92.08,63.25 | 93.98,67.69 92.08,67.69 92.08,67.44 94.11,67.44 94.11,67.31 94.23,67.31 94.23,67.82 91.95,67.82 91.95,67.69 91.82,67.69 91.82,67.18 94.36,67.18 94.36,67.94 U$18.7 U$18.6
  Top 0.61: 92.84,63.12 93.73,63.12 93.85,63.25
  Top 0.813: 91.95,67.82 91.95,67.44 | 96.14,65.79 96.24,65.79 96.65,65.38
  Top 1.016: 91.95,67.44 95.38,67.44 96.14,66.67 96.14,65.79 96.14,64.01 95.38,63.25 93.85,63.25
  Top 1.27: 96.65,65.38 v97.81,65.38
  Bottom 1.27: v97.81,65.38 97.81,67.36 100.05,69.6 107.16,69.6 108.43,70.87 108.43,104.7 103.35,109.78 U$17.50
VR1+
  Top 0.254: 89.6,95.96 R29.1
  Top 0.305: 89.66,96.26 R29.1
  Top 0.406: 89.6,95.96 R25.2 | 89.66,96.26 91.56,96.26 92.33,97.03 92.33,110.91 U$17.47
VR1-
  Top 0.406: R26.2 95.38,90.99 R29.2 94.23,96.14 93.22,97.16 93.22,105.92 96.65,109.35 96.65,111.89 U$17.48
VR2+
  Top 0.254: 105.47,95.69 104.97,95.69
  Top 0.305: 104.78,95.5 104.97,95.69 R32.2
  Top 0.406: 105.47,95.69 R27.2 | R32.2 105.42,99.95 108.38,102.92 108.38,115.11 U$17.38
VR2-
  Top 0.406: R56.2 99.82,90.73 R32.1 102.36,96.14 103.5,97.28 103.5,100.99 105.08,102.56 105.08,115.14 U$17.37
(copper drawn outside any net)
  shapes: Bottom area x15

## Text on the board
tNames: HALL2 | GND | GND | VR2- | VR2+ | SDA | SCL | HC2 | INJ1 | LC1 | TACHO | FAN | FUEL | IAT | CLT | IGN4 | CAN H | CAN L | TPS | RX | TX | RX5 | TX5 | UD- | UD+ | O2_2 | CLUTCH | HC1 | 1A | 1B | 2A | 2B | O2 | INJ3 | INJ6 | VIN | INJ8 | INJ7 | IDLE | INJ2 | INJ5 | INJ4 | IGN5 | IGN6 | IGN7 | IGN8 | IGN3 | IGN1 | IGN2 | VR1+ | VR1- | +5V_2 | +12V | HALL1 | BOOST | MAP_EXT | STEPPER DRIVER | INJ6 | INJ7 | STP | DIR | IGN3 | IGN4 | IGN1 | IGN2 | INJ8 | INJ5 | CRANK | CAM | IGN5 | IGN6 | IGN7 | IGN8 | GND | BOOST | FUEL | 47 | +5V | 48 | INJ4 | FAN | 49 | Designed for Speeduino firmware | 50 | TACHO | 51 | IDLE | 52 | INJ3 | 53 | GND | LC1 | 3V3 | HC2 | . | INJ2 | Author: Krzysztof Dymianiuk@ Seaside Customs Garage | . | HC1 | SCG-ECU 1.0 | INJ1 | 20191125
bStop: SCG-ECU | *** | 1.0 | *** | SEASIDE CUSTOMS | GARAGE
